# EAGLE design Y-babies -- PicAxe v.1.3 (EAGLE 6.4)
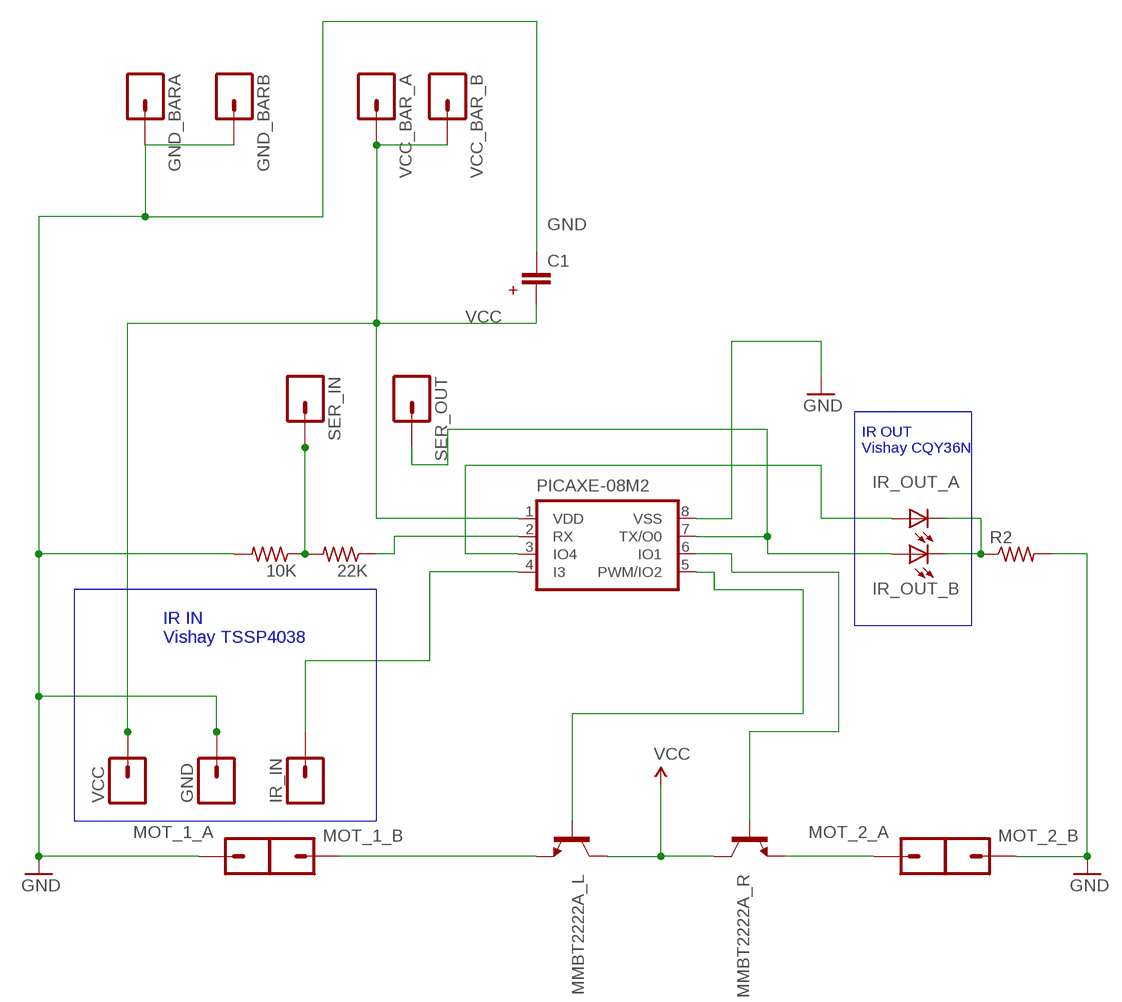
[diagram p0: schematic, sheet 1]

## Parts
10K  R-US_R0805W  [R0805W]
22K  R-US_R0805W  [R0805W]
C1  CAPPTH1  [CAP-PTH-5MM]
GND  M01PTH  [1X01]
GND_BARA  M01PTH  [1X01]
GND_BARB  M01PTH  [1X01]
IR_IN  M01PTH  [1X01]
IR_OUT_A  LED3MM  [LED3MM]
IR_OUT_B  LED3MM  [LED3MM]
MMBT2222A_L  TRANSISTOR_NPNSOT23  [SOT23]
MMBT2222A_R  TRANSISTOR_NPNSOT23  [SOT23]
MOT_1_A  M01SMD-4.5X1.5  [PAD-1.5X4.5]
MOT_1_B  M01SMD-4.5X1.5  [PAD-1.5X4.5]
MOT_2_A  M01SMD-4.5X1.5  [PAD-1.5X4.5]
MOT_2_B  M01SMD-4.5X1.5  [PAD-1.5X4.5]
PICAXE-08M2  PICAXE-08M2  PICAXE-08M  [DIL8]
R2  R-US_R0805W  [R0805W]
SER_IN  M01PTH  [1X01]
SER_OUT  M01PTH  [1X01]
VCC  M01PTH  [1X01]
VCC_BAR_A  M01PTH  [1X01]
VCC_BAR_B  M01PTH  [1X01]

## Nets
GND: 10K.2 C1.1 GND.1 GND_BARA.1 GND_BARB.1 MOT_1_A.P$1 MOT_2_B.P$1 PICAXE-08M2.8(VSS) R2.2
N$1: MMBT2222A_L.1(B) PICAXE-08M2.5(PWM/IO2)
N$2: MMBT2222A_R.1(B) PICAXE-08M2.6(IO1)
N$3: IR_OUT_B.A PICAXE-08M2.7(TX/O0) SER_OUT.1
N$5: 10K.1 22K.2 SER_IN.1
N$6: IR_OUT_A.A PICAXE-08M2.3(IO4)
N$7: IR_OUT_A.K(C) IR_OUT_B.K(C) R2.1
N$8: 22K.1 PICAXE-08M2.2(RX)
N$9: MMBT2222A_L.2(E) MOT_1_B.P$1
N$10: MMBT2222A_R.2(E) MOT_2_A.P$1
N$11: IR_IN.1 PICAXE-08M2.4(I3)
VCC: C1.2 MMBT2222A_L.3(C) MMBT2222A_R.3(C) PICAXE-08M2.1(VDD) VCC.1 VCC_BAR_A.1 VCC_BAR_B.1

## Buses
B$1
B$2

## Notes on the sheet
- +
- IR OUT
  Vishay CQY36N
- IR IN
  Vishay TSSP4038

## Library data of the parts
10K 22K R2 = resistor:R-US_: RESISTOR, American symbol
C1 = SparkFun:CAP: Capacitor
GND GND_BARA GND_BARB IR_IN MOT_1_A MOT_1_B MOT_2_A MOT_2_B SER_IN SER_OUT VCC VCC_BAR_A VCC_BAR_B = SparkFun:M01: Header 1
IR_OUT_A IR_OUT_B = led:LED: LED
MMBT2222A_L MMBT2222A_R = SparkFun:TRANSISTOR_NPN: Transistor NPN BJT configuration in SOT23 package. MMBT2222 is the common NPN we use. Double check BCE configuration again layout.
PICAXE-08M2 = picaxe-3:PICAXE-08M

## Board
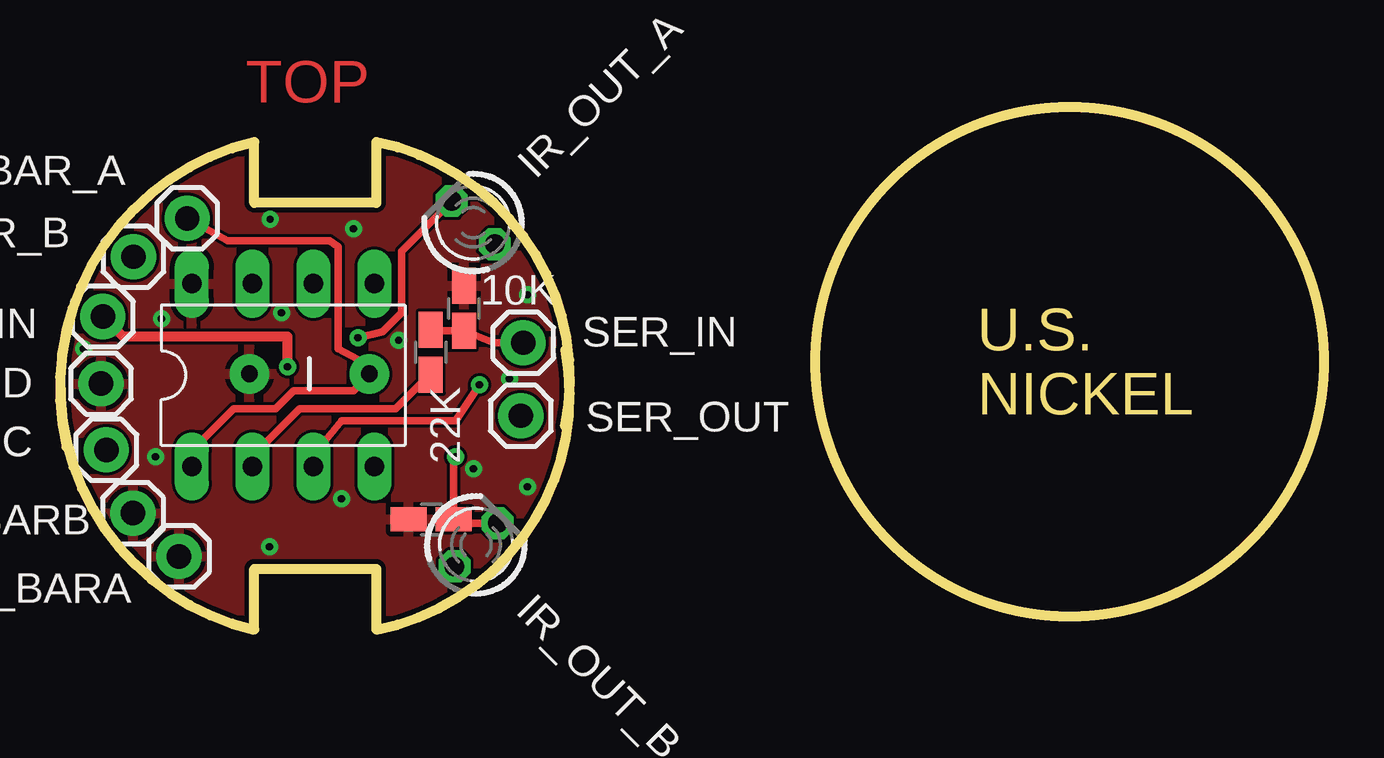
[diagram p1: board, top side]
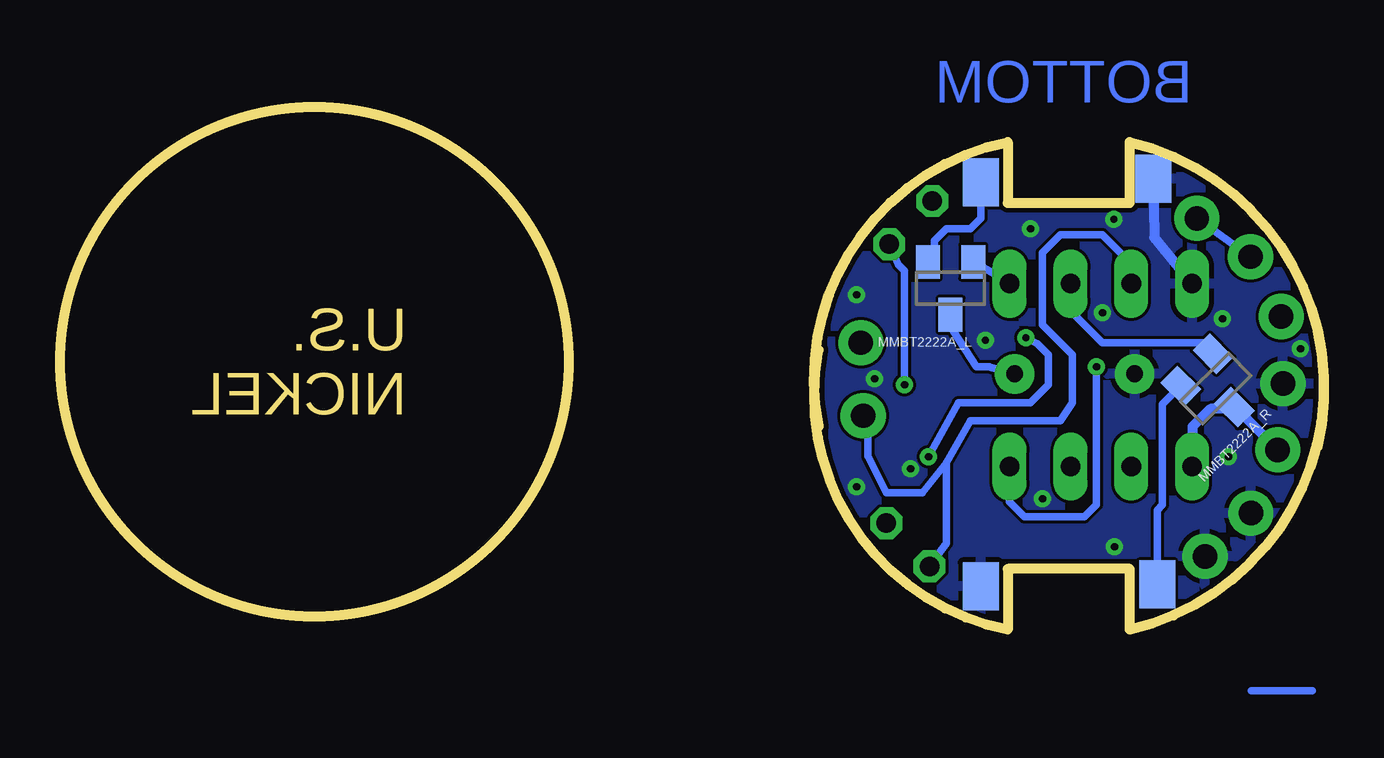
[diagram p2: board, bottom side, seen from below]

Size 52.69 x 21.77 mm. Coordinates in mm from the lower left corner, seen from the top.
Outline: 0.27,7.62 arc-90 8.1,20.32 8.1,17.78 13.18,17.78 13.18,20.32 arc-90 21.06,8.46
Outline: 0.27,12.48 arc90 8.1,0 8.1,2.54 13.18,2.54 13.18,0 arc90 21.07,11.66
Outline: circle at 42.08,11.16 radius 10.61
Copper layers (1*16): Top 0.035mm / dielectric 1.5mm / Bottom 0.035mm
Design rules "default *": minimum track width 10mil, minimum drill 24mil, track to track 5mil, track to pad 5mil, pad to pad 5mil, via to via 5mil, smd to smd 5mil, copper to edge 8mil, drill to drill 6mil, minimum pad ring 10mil, minimum via ring 8mil, stop-mask expansion 4mil, vias tented up to drill 0.3mm, thermal gap 8mil

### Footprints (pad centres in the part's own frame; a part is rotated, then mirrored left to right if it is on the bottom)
R0805W = smd 1.5 x 1: 1 -0.94,0; 2 0.94,0
CAP-PTH-5MM = drill 0.7 pad 1.651: 1 -2.5,0; 2 2.5,0
1X01 = drill 1.016 pad 1.88: 1 0,0
LED3MM = drill 0.813 octagon: A -1.27,0; K 1.27,0
SOT23 = smd 1 x 1.4: 1 -0.95,-1.1; 2 0.95,-1.1; 3 0,1.1
PAD-1.5X4.5 = smd 1.5 x 2: P$1 0,0
DIL8 = drill 0.813 pad 1.422 long: 1 -3.81,-3.81; 2 -1.27,-3.81; 3 1.27,-3.81; 4 3.81,-3.81; 5 3.81,3.81; 6 1.27,3.81; 7 -1.27,3.81; 8 -3.81,3.81

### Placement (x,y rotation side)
10K  16.84,13.39 90 top
22K  15.46,11.56 90 top
C1  10.39,10.66 0 top
GND  1.71,10.26 0 top
GND_BARA  4.96,3.05 0 top
GND_BARB  3.04,4.86 0 top
IR_IN  1.79,13.05 0 top
IR_OUT_A  17.22,16.96 135 top
IR_OUT_B  17.34,3.54 45 top
MMBT2222A_L  15.57,14.22 180 bottom
MMBT2222A_R  4.51,10.05 225 bottom
MOT_1_A  7.12,18.78 0 bottom
MOT_1_B  14.29,18.65 180 bottom
MOT_2_A  6.96,1.89 180 bottom
MOT_2_B  14.31,1.81 0 bottom
PICAXE-08M2  9.3,10.61 0 top
R2  15.48,4.6 180 top
SER_IN  19.31,11.96 0 top
SER_OUT  19.21,8.92 0 top
VCC  1.93,7.49 0 top
VCC_BAR_A  5.3,17.14 0 top
VCC_BAR_B  3.06,15.54 0 top

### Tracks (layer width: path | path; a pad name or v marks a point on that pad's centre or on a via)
GND  (via drill 0.3)
  Bottom 0.406: MOT_1_A.P$1 7.08,16.35 PICAXE-08M2.8
  other vias: 8.73,3.46 0.98,11.71 19.48,5.96 12.23,16.71 19.48,13.96 4.23,12.96 8.76,17.11 11.73,5.46 3.98,7.21 18.73,10.46 17.23,6.71 14.11,12.06 9.23,13.21
  pour Bottom: -0.79,20.32 -0.79,0 22.07,0 22.07,20.32
  pour Top: -0.79,20.32 -0.79,0 22.07,0 22.07,20.32
N$1
  Bottom 0.305: MMBT2222A_L.1 13.71,14.81 PICAXE-08M2.5
N$2
  Bottom 0.305: PICAXE-08M2.6 10.57,13.3 9.23,11.96 5.08,11.96 MMBT2222A_R.1
N$3
  Bottom 0.305: PICAXE-08M2.7 8.03,15.26 9.23,16.46 10.98,16.46 11.73,15.71 11.73,12.71 10.48,11.46 10.48,9.46 10.98,8.71 14.73,8.71 15.73,6.96 | SER_OUT.1 19,8.71 19,7.23 18.23,5.71 16.73,5.71 15.73,6.96 | 15.73,6.96 15.73,3.6 IR_OUT_B.A
N$4
  Bottom 0.305: 0.48,-2.54 3.02,-2.54
N$5
  Top 0.305: SER_IN.1 18.08,11.95 10K.1 15.51,12.45 22K.2
N$6  (via drill 0.3)
  Top 0.305: PICAXE-08M2.3 10.57,7.3 11.73,8.71 16.48,8.71 v17.48,10.21
  Bottom 0.305: v17.48,10.21 17.48,14.96 17.73,15.2 IR_OUT_A.A
N$7  (via drill 0.3)
  Top 0.305: IR_OUT_B.K 16.58,4.44 R2.1 16.42,6.89 v16.48,7.21 | v12.42,12.17 13.44,12.42 14.23,13.21 14.23,15.77 IR_OUT_A.K
  Bottom 0.305: v12.42,12.17 11.94,11.92 11.48,11.46 11.48,10.21 12.23,9.46 15.23,9.46 v16.48,7.21
N$8
  Top 0.305: PICAXE-08M2.2 8.03,7.26 9.98,9.21 13.98,9.21 15.23,10.46 15.3,10.46 22K.1
N$9
  Bottom 0.305: MOT_1_B.P$1 14.29,17.15 14.73,16.71 15.73,16.71 16.23,16.21 16.23,15.61 MMBT2222A_L.2
N$10
  Bottom 0.305: MOT_2_A.P$1 6.96,4.99 6.73,5.21 6.73,9.39 MMBT2222A_R.2
N$11  (via drill 0.3)
  Top 0.406: v9.48,10.96 9.48,12.21 2.63,12.21 IR_IN.1
  Bottom 0.305: PICAXE-08M2.4 13.11,5.33 12.48,4.71 9.98,4.71 9.48,5.21 v9.48,10.96
VCC
  Top 0.305: 12.98,10.71 12.98,10.96 11.59,11.71 11.59,15.96 11.23,16.21 6.98,16.21 VCC_BAR_A.1 | 5.48,7.46 7.23,9.21 8.98,9.21 9.73,9.96 12.23,9.96 12.98,10.71 | 12.98,10.71 12.94,10.71 C1.2
  Top 0.406: PICAXE-08M2.1 5.49,7.45 5.48,7.46
  Bottom 0.305: MMBT2222A_L.3 15.45,12.43 14.48,10.96 13.98,10.96 | 13.98,10.96 13.94,10.96 | C1.2 12.93,10.66 13.98,10.96 | VCC_BAR_A.1 VCC_BAR_B.1 2.73,14.84 | MMBT2222A_R.3 3.74,9.2
  Bottom 0.406: VCC.1 3.64,9.2 3.74,9.2 4.74,9.2 5.48,8.46 PICAXE-08M2.1

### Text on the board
Top: TOP
Bottom: BOTTOM
Dimension: U.S. / NICKEL

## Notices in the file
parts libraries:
SparkFun: Licensing: CC v3.0 Share-Alike You are welcome to use this library for commercial purposes.
